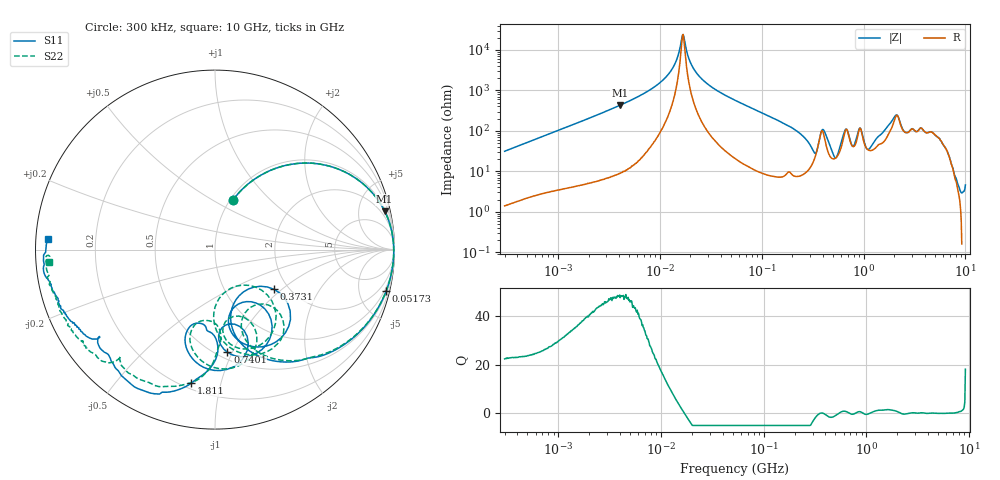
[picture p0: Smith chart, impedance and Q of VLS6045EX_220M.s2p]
! S-Parameter Data Generated by TDK Corporation
! Copyright(C) 2019 TDK Corporation.
! All Rights Reserved.
! TDK P/N: VLS6045EX-220M (Inductor)
! Property: L=22uH at 100kHz
! Size(LxWxT): 6x6x4.5mm
! Model Type: s2p (Touchstone File Format Version 1.0)
! Frequency: DC=Yes Start=0.3MHz Stop=10000MHz 802points Log-sweep
! Model Generated on May 10, 2019
! Port Assignments:
!  1 ---@@@--- 2
! Applicable Conditions:
!  Temperature = 25 degC
!  DC Bias Current = 0 A
!  Small Signal Operation
! Terms and conditions regarding TDK Simulation Models
! (1)This simulation model is being provided solely for informational purposes. Please refer to the specifications of the products in terms of detailed characteristics of such products.
! (2)In no event shall TDK Corporation of any of its subsidiaries be liable for any loss or damage arising, directly or indirectly,
!  From any information contained in this simulation model, including, but not limited to loss or damages arising from any inaccuracies, omissions or errors in connection with such information.
! (3)Any and all copyrights on this simulation model are owned by TDK Corporation.
!  Duplication or redistribution of this simulation model without prior written permission from TDK Corporation is prohibited.
! (4)This simulation model is subject to any modification or change without any prior notice.
! (5)Neither TDK Corporation nor any of its subsidiaries shall make any warranty, express or implied,
!  Including but not limited to the correctness, implied warranties of merchantability and fitness for a particular purpose with respect to this simulation models.
! (6)The use of this simulation model shall be deemed to have consented to the terms and conditions hereof.
# Hz S MA R 50
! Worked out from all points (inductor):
!   801 points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, 300 kHz to 10 GHz, reference 50 ohm
!   read as one part in series: L = 16.4 uH near 318.3 kHz
!   highest Q = 48.4 at 4.054 MHz (marker M1), where L = 16.8 uH
!   self-resonance near 16.72 MHz
!   S11 on the Smith chart (normalised r, x): 300 kHz: 1.03, +0.62; 51.73 MHz: 0.66, -8.29; 373.1 MHz: 1.68, -0.88; 740.1 MHz: 0.56, -0.96; 1.811 GHz: 0.23, -0.81; 10 GHz: 0.03, +0.03
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300000  0.2929 70.3  0.9429 -17.2  0.9431 -17.2  0.2928 70.2
1713600  0.8558 29.5  0.4953 -59.0  0.4954 -59.0  0.8557 29.5
4053600  0.9691 12.8  0.2273 -76.0  0.2272 -76.0  0.9692 12.8
9671944  0.9938 3.1  0.06925 -83.8  0.06928 -83.8  0.994 3.2
1.35567e7  0.9956 0.3  0.02645 -81.1  0.02647 -81.1  0.9958 0.4
1.694973e7  0.9958 -1.5  0.00412 3.5  0.004104 3.2  0.996 -1.4
2.378472e7  0.9947 -4.4  0.04125 79.5  0.04126 79.5  0.9949 -4.3
5.172916e7  0.9813 -13.7  0.1591 74.3  0.1591 74.3  0.9814 -13.4
5.477226e7  0.9792 -14.6  0.1703 73.5  0.1703 73.5  0.9794 -14.3
1.720721e8  0.8234 -46.6  0.5221 41.0  0.522 41.0  0.828 -45.4
3.126428e8  0.4523 -77.6  0.7718 0.7  0.7718 0.7  0.4812 -71.7
3.730642e8  0.395 -34.0  0.5647 -24.2  0.5647 -24.2  0.4852 -44.4
4.448526e8  0.5911 -66.6  0.6111 -2.2  0.611 -2.2  0.5935 -76.0
5.82867e8  0.3311 -62.7  0.7257 -39.5  0.7256 -39.5  0.2325 -67.0
6.573376e8  0.5603 -55.7  0.4582 -51.6  0.4582 -51.6  0.5 -47.1
7.400828e8  0.576 -83.1  0.5234 -31.7  0.5234 -31.7  0.5512 -78.7
1.260284e9  0.4192 -101.7  0.5801 -79.4  0.581 -79.4  0.3976 -97.1
1.767019e9  0.728 -98.1  0.2471 -132.5  0.248 -132.6  0.759 -101.0
1.810952e9  0.7549 -100.0  0.2224 -134.2  0.2233 -134.3  0.7775 -103.8
2.142542e9  0.8824 -117.5  0.092 -109.7  0.0926 -110.2  0.8374 -121.6
2.629198e9  0.8428 -133.7  0.1573 -105.9  0.1571 -106.5  0.7943 -131.5
1e10  0.9345 176.5  0.04538 -151.5  0.0454 -151.4  0.9256 -175.7
